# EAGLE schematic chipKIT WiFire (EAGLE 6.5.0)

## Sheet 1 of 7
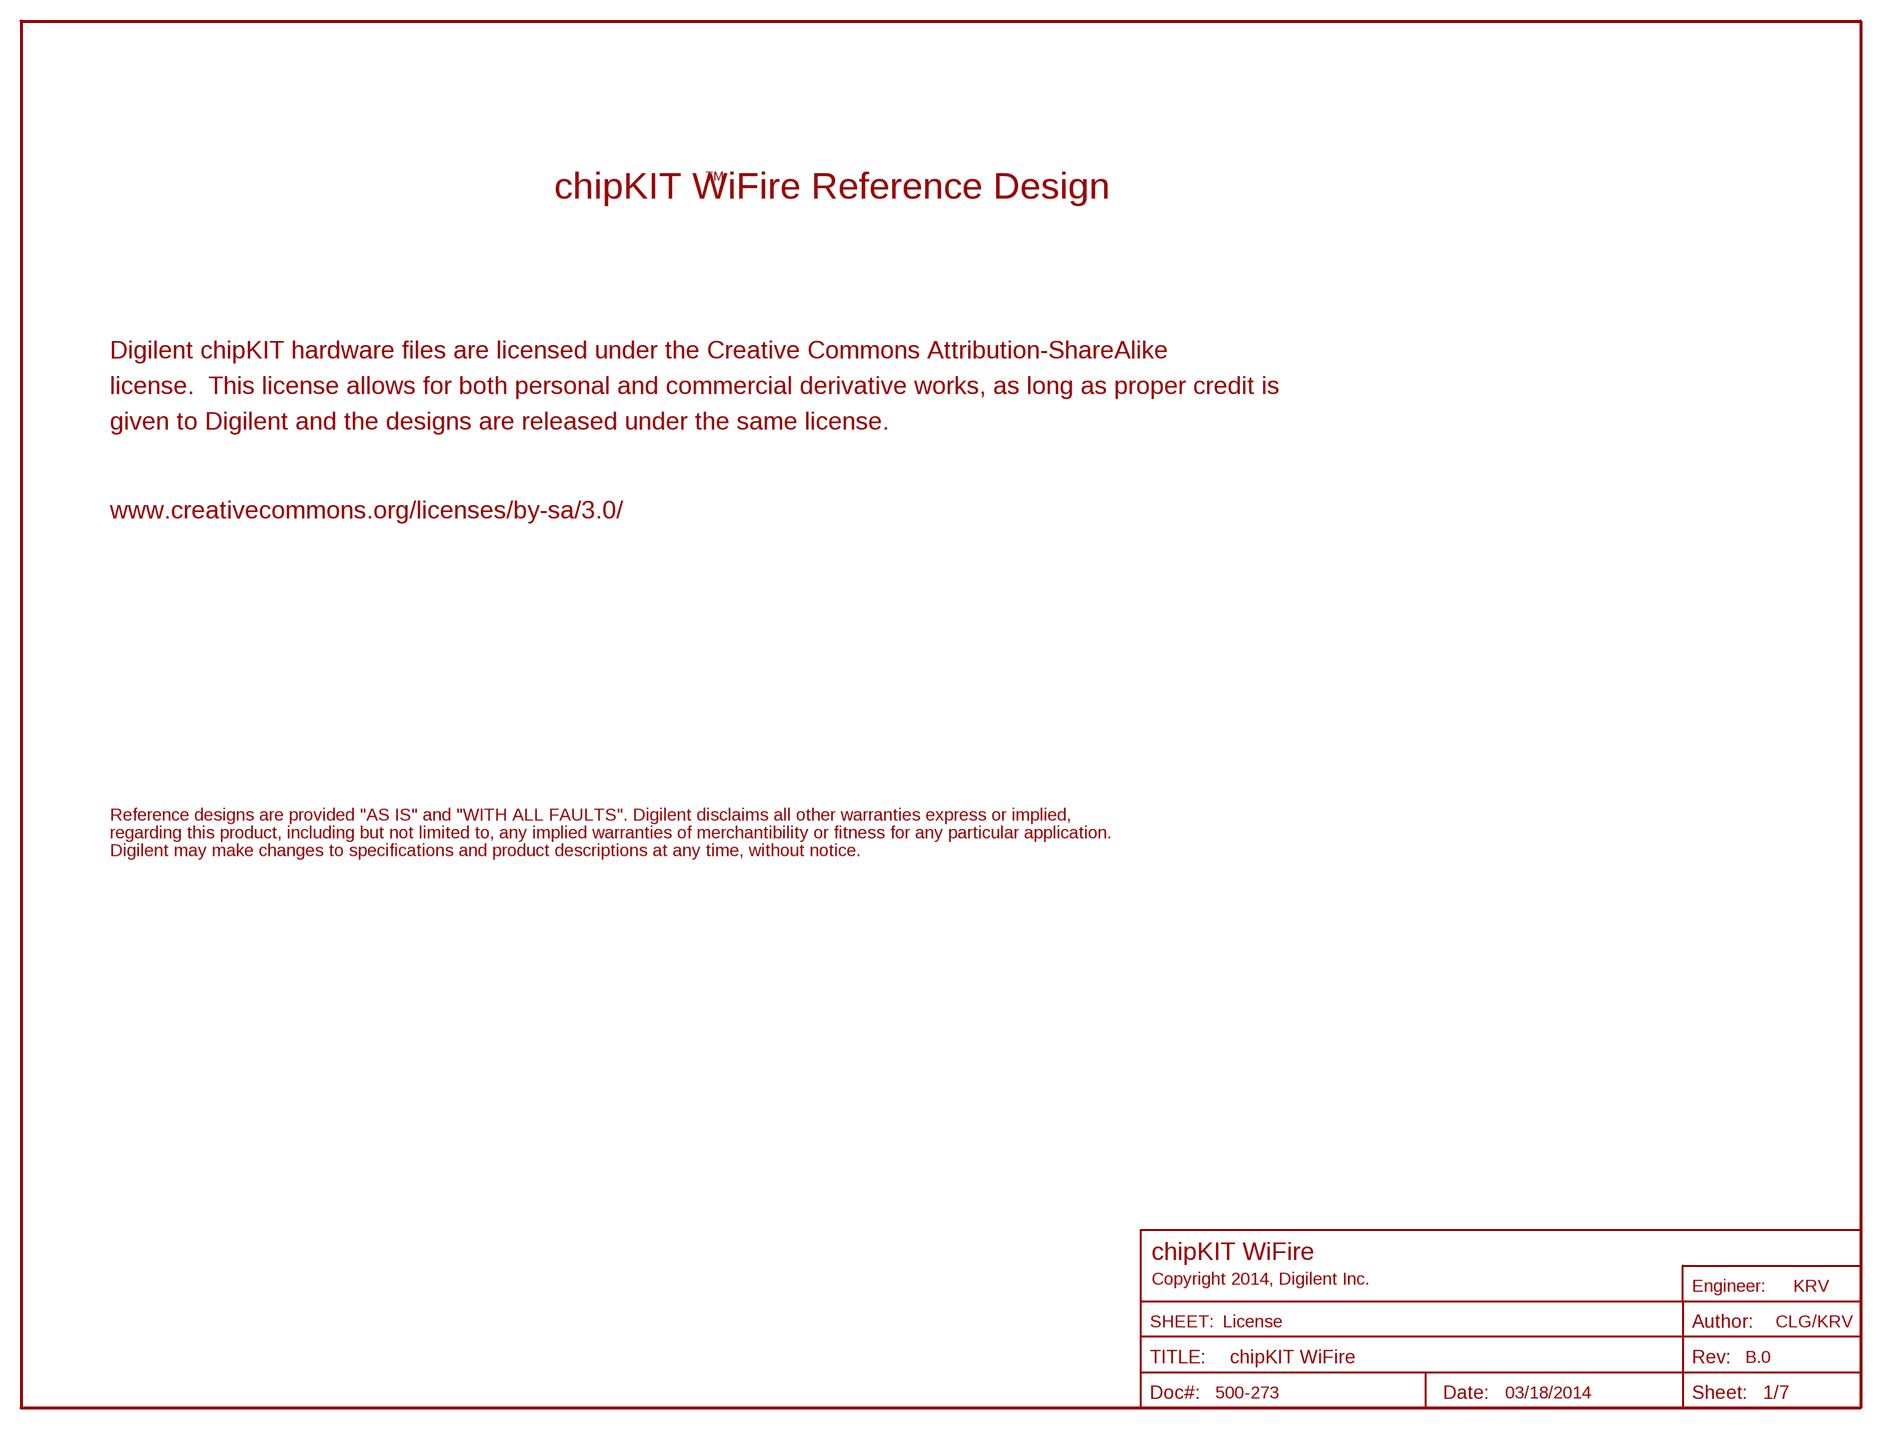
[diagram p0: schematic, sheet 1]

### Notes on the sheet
- TM
- chipKIT WiFire Reference Design
- Digilent chipKIT hardware files are licensed under the Creative Commons Attribution-ShareAlike
- license.  This license allows for both personal and commercial derivative works, as long as proper credit is
- given to Digilent and the designs are released under the same license.
- www.creativecommons.org/licenses/by-sa/3.0/
- Reference designs are provided "AS IS" and "WITH ALL FAULTS". Digilent disclaims all other warranties express or implied,
- regarding this product, including but not limited to, any implied warranties of merchantibility or fitness for any particular application.
- Digilent may make changes to specifications and product descriptions at any time, without notice.
- chipKIT WiFire
- Copyright 2014, Digilent Inc.
- KRV
- License | CLG/KRV
- B.0
- 500-273 | 03/18/2014

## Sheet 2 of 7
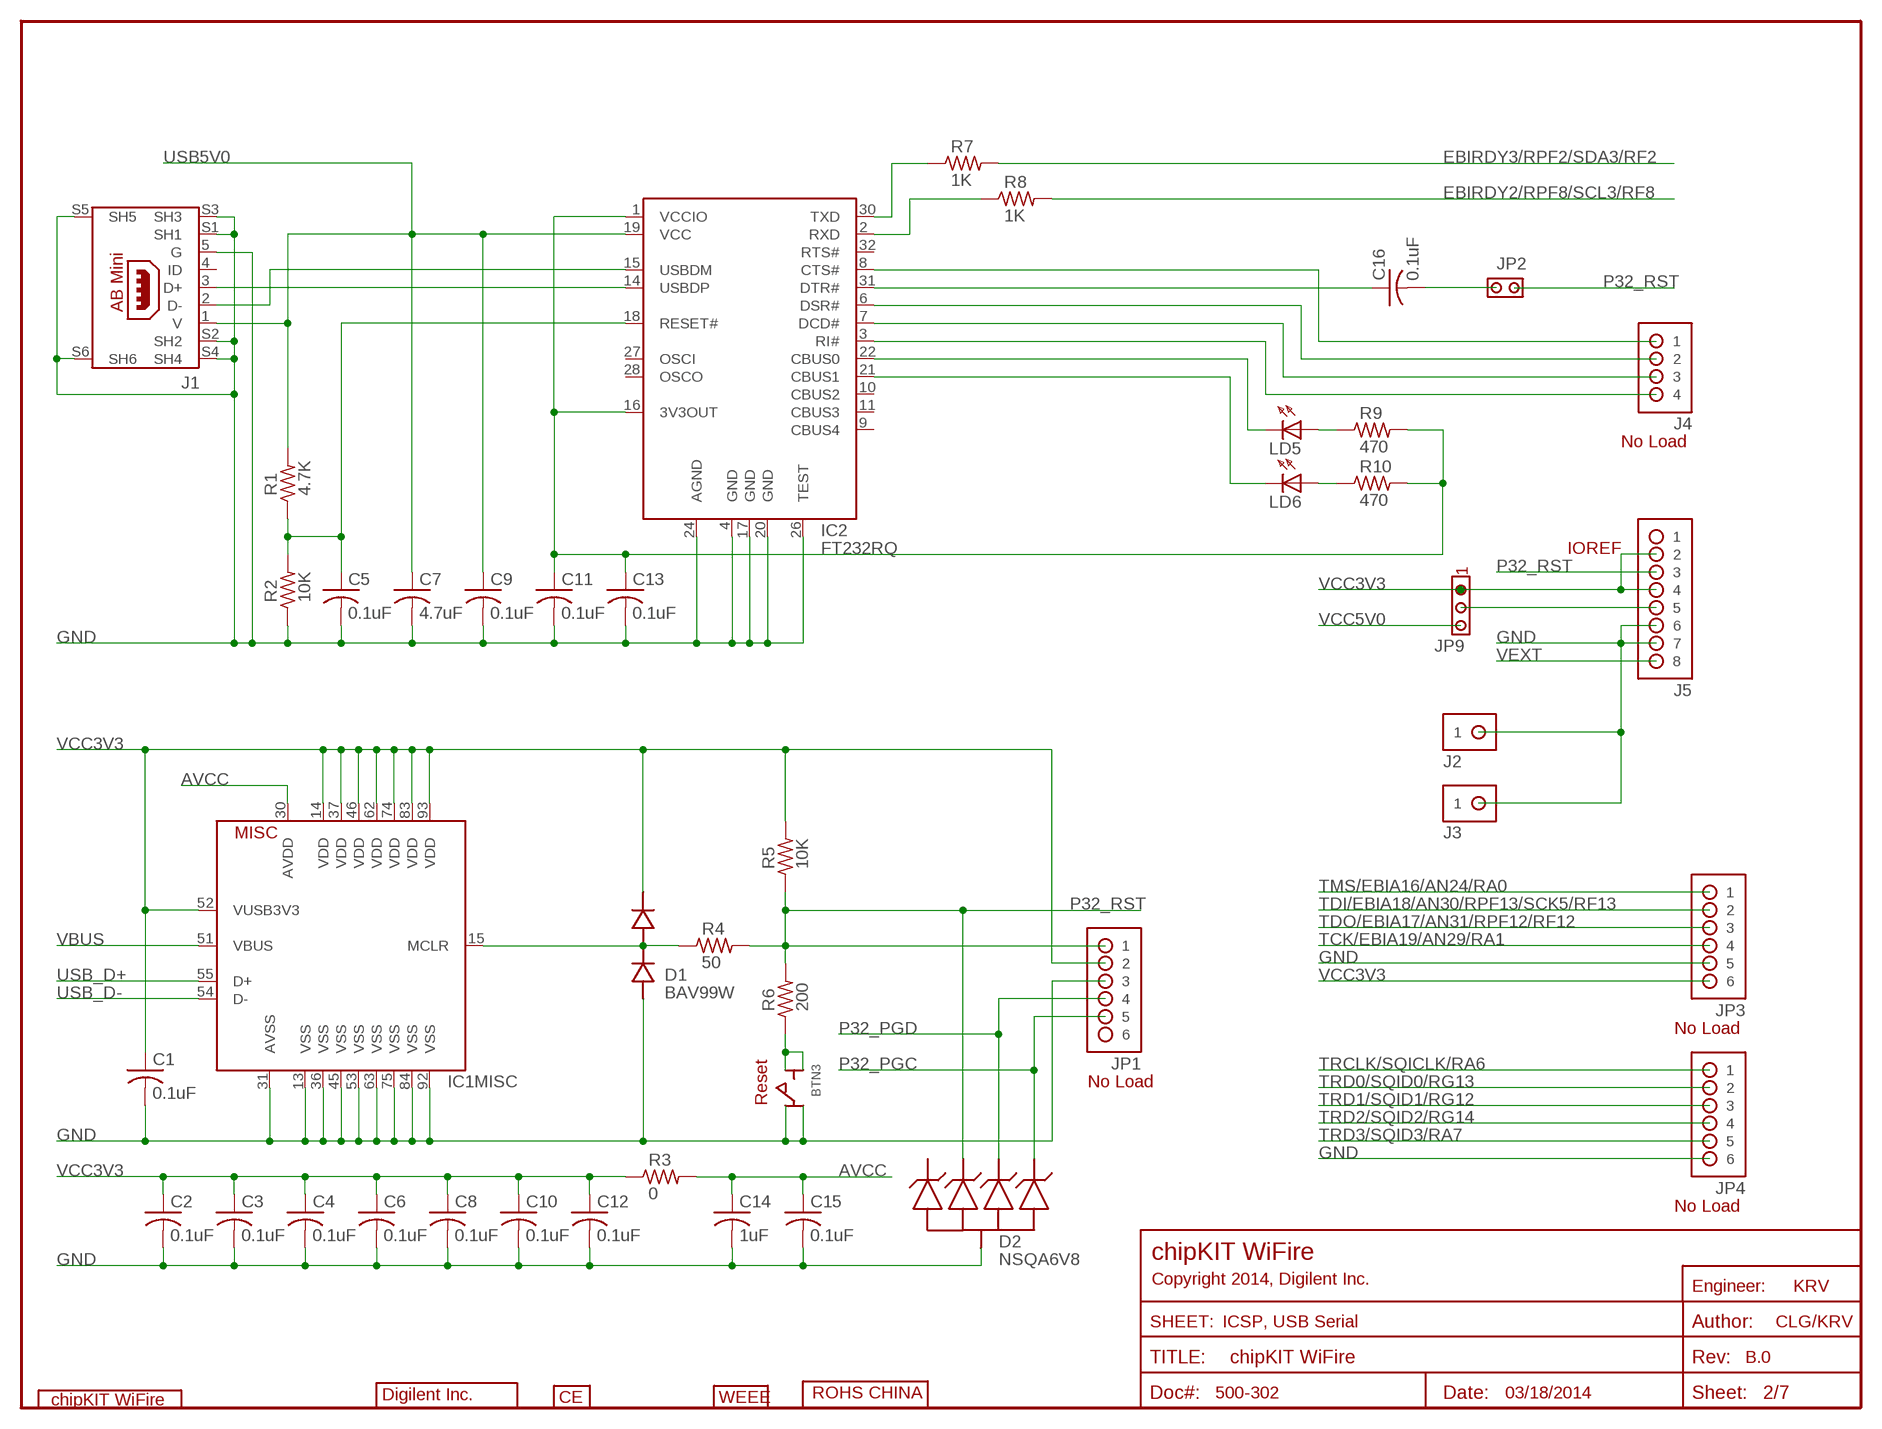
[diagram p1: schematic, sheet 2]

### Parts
BTN3  SW-P8008  [SW-P8008]
C1  0.1uF  CAP-S0402S  [C0402S]
C2  0.1uF  CAP-S0402S  [C0402S]
C3  0.1uF  CAP-S0402S  [C0402S]
C4  0.1uF  CAP-S0402S  [C0402S]
C5  0.1uF  CAP-S0402S  [C0402S]
C6  0.1uF  CAP-S0402S  [C0402S]
C7  4.7uF  CAP-S0603S  [C0603S]
C8  0.1uF  CAP-S0402S  [C0402S]
C9  0.1uF  CAP-S0402S  [C0402S]
C10  0.1uF  CAP-S0402S  [C0402S]
C11  0.1uF  CAP-S0402S  [C0402S]
C12  0.1uF  CAP-S0402S  [C0402S]
C13  0.1uF  CAP-S0402S  [C0402S]
C14  1uF  CAP-S0402S  [C0402S]
C15  0.1uF  CAP-S0402S  [C0402S]
C16  0.1uF  CAP-S0402S  [C0402S]
D1  BAV99W  [SOT-323]
D2  NSQA6V8  [SOT-323-5]
IC1  PIC32MZ2048ECG100-PT  PIC32MZECX100-PT  [TQ100-PT]
IC2  FT232RQ  [QFN32]
J1  KMAB-SMT-5S  USB-AB-MINI  [USB-AB-MINI]
J2  ST. Male  HDR-1X1  [HDR-1X1]
J3  ST. Male  HDR-1X1  [HDR-1X1]
J4  No Load  HDR-1X4  [HDR-1X4]
J5  ST. Female  HDR-1X8  [HDR-1X8]
JP1  No Load  HDR-1X6-OFFSET  [HDR-1X6_OFFSET]
JP2  ST. Male  JPR-1X2  [JPR-1X2]
JP3  No Load  HDR-1X6-OFFSET  [HDR-1X6_OFFSET]
JP4  No Load  HDR-1X6-OFFSET  [HDR-1X6_OFFSET]
JP9  JPR-1X3  [JPR-1X3]
LD5  Red  LED-S0603S  [D0603S]
LD6  Red  LED-S0603S  [D0603S]
LOGO1  DIGILENT_INC-BT-1000  [DIGILENT_BEYOND_1000_LOGO]
LOGO2  CE  [CE_LOGO]
LOGO3  WEEE-S  [WEEE_LOGO]
LOGO4  ROHS-CHINA  [ROHS_CHINA_LOGO]
R1  4.7K  RES-S0402S  [R0402S]
R2  10K  RES-S0402S  [R0402S]
R3  0  RES-S0603S  [R0603S]
R4  50  RES-S0402S  [R0402S]
R5  10K  RES-S0402S  [R0402S]
R6  200  RES-S0402S  [R0402S]
R7  1K  RES-S0402S  [R0402S]
R8  1K  RES-S0402S  [R0402S]
R9  470  RES-S0402S  [R0402S]
R10  470  RES-S0402S  [R0402S]
U$1  CHIPKIT_WIFIRE_LOGO  [CHIPKIT_WIFIRE_LOGO]

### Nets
AVCC: C14.1 C15.1 IC1.30(MISC:AVDD) R3.2
EBIRDY2/RPF8/SCL3/RF8: R8.2 ; also sheet 3,5
EBIRDY3/RPF2/SDA3/RF2: R7.2 ; also sheet 3,5
FT3V3: C11.1 C13.1 IC2.1(VCCIO) IC2.16(3V3OUT) R9.2 R10.2
GND: BTN3.1A BTN3.2A C1.2 C2.2 C3.2 C4.2 C5.2 C6.2 C7.2 C8.2 C9.2 C10.2 C11.2 C12.2 C13.2 C14.2 C15.2 D1.1(CAT) D2.2(COM) IC1.13(MISC:VSS) IC1.31(MISC:AVSS) IC1.36(MISC:VSS) IC1.45(MISC:VSS) IC1.53(MISC:VSS) IC1.63(MISC:VSS) IC1.75(MISC:VSS) IC1.84(MISC:VSS) IC1.92(MISC:VSS) IC2.4(GND) IC2.17(GND) IC2.20(GND) IC2.24(AGND) IC2.26(TEST) J1.5(G) J1.S1(SH1) J1.S2(SH2) J1.S3(SH3) J1.S4(SH4) J1.S5(SH5) J1.S6(SH6) J2.1 J3.1 J5.6 J5.7 JP1.3 JP3.5 JP4.6 R2.1 ; also sheet 3,4,5,6,7
N$14: C16.2 JP2.2
N$21: D1.3(COM) IC1.15(MISC:MCLR) R4.1
N$27: BTN3.1B BTN3.2B R6.1
N$33: IC2.15(USBDM) J1.2(D-)
N$37: IC2.14(USBDP) J1.3(D+)
N$41: IC2.30(TXD) R7.1
N$43: IC2.2(RXD) R8.1
N$47: C5.1 IC2.18(RESET#) R1.1 R2.2
N$52: IC2.8(CTS#) J4.1
N$53: C16.1 IC2.31(DTR#)
N$54: IC2.6(DSR#) J4.2
N$55: IC2.7(DCD#) J4.3
N$56: IC2.3(RI#) J4.4
N$57: IC2.22(CBUS0) LD5.C
N$58: IC2.21(CBUS1) LD6.C
N$59: LD5.A R9.1
N$60: LD6.A R10.1
P32_PGC: D2.5(D4) JP1.5 ; also sheet 4
P32_PGD: D2.4(D3) JP1.4 ; also sheet 4
P32_RST: D2.3(D2) J5.3 JP1.1 JP2.1 R4.2 R5.1 R6.2
TCK/EBIA19/AN29/RA1: JP3.4 ; also sheet 4
TDI/EBIA18/AN30/RPF13/SCK5/RF13: JP3.2 ; also sheet 5
TDO/EBIA17/AN31/RPF12/RF12: JP3.3 ; also sheet 5
TMS/EBIA16/AN24/RA0: JP3.1 ; also sheet 4
TRCLK/SQICLK/RA6: JP4.1 ; also sheet 4
TRD0/SQID0/RG13: JP4.2 ; also sheet 5
TRD1/SQID1/RG12: JP4.3 ; also sheet 5
TRD2/SQID2/RG14: JP4.4 ; also sheet 5
TRD3/SQID3/RA7: JP4.5 ; also sheet 4
USB5V0: C7.1 C9.1 IC2.19(VCC) J1.1(V) R1.2 ; also sheet 7
USB_D+: IC1.55(MISC:D+) ; also sheet 6
USB_D-: IC1.54(MISC:D-) ; also sheet 6
VBUS: IC1.51(MISC:VBUS) ; also sheet 6,7
VCC3V3: C1.1 C2.1 C3.1 C4.1 C6.1 C8.1 C10.1 C12.1 D1.2(AN) IC1.14(MISC:VDD) IC1.37(MISC:VDD) IC1.46(MISC:VDD) IC1.52(MISC:VUSB3V3) IC1.62(MISC:VDD) IC1.74(MISC:VDD) IC1.83(MISC:VDD) IC1.93(MISC:VDD) J5.2 J5.4 JP1.2 JP3.6 JP9.1 R3.1 R5.2 ; also sheet 4,5,6,7
VCC5V0: JP9.3 ; also sheet 6,7
VCCSHIELD: J5.5 JP9.2
VEXT: J5.8 ; also sheet 7
Unconnected: D2.1(D1) IC2.9(CBUS4) IC2.10(CBUS2) IC2.11(CBUS3) IC2.27(OSCI) IC2.28(OSCO) IC2.32(RTS#) J1.4(ID) J5.1 JP1.6

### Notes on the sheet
- No Load
- IOREF
- No Load
- No Load
- Reset
- No Load
- chipKIT WiFire
- Copyright 2014, Digilent Inc.
- KRV
- ICSP, USB Serial | CLG/KRV
- B.0
- 500-302 | 03/18/2014

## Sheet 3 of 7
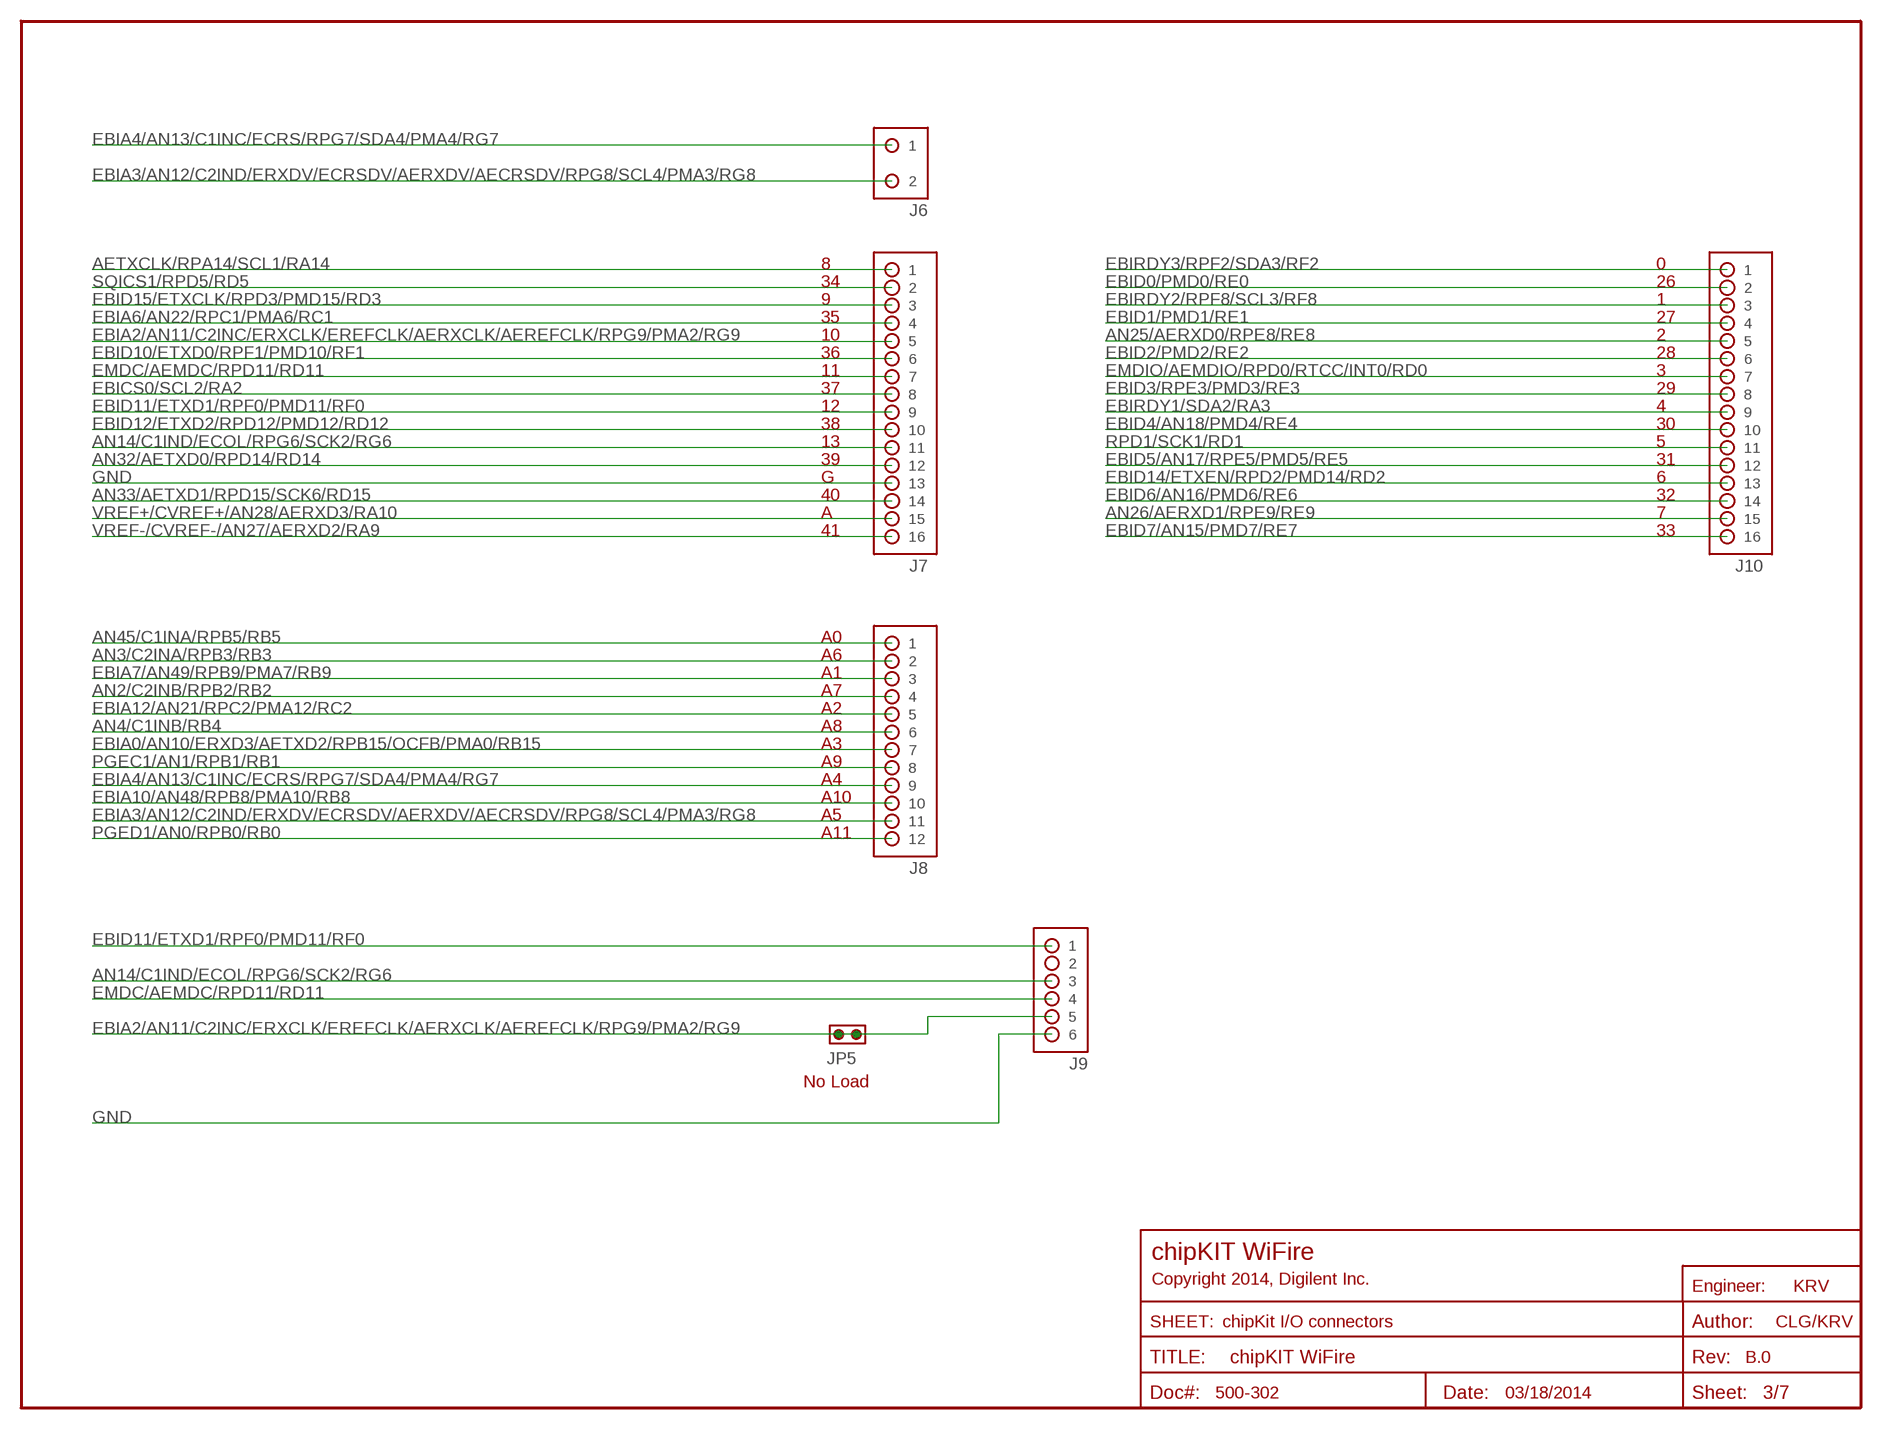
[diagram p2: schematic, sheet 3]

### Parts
J6  ST. Female  HDR-1X2  [HDR-1X2]
J7  ST. Female  HDR-2X8  [HDR-2X8]
J8  ST. Female  HDR-2X6  [HDR-2X6]
J9  ST. Male  HDR-2X3  [HDR-2X3]
J10  ST. Female  HDR-2X8  [HDR-2X8]
JP5  No Load  JPR-1X2  [JPR-1X2]

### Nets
AETXCLK/RPA14/SCL1/RA14: J7.1 ; also sheet 4,6
AN2/C2INB/RPB2/RB2: J8.4 ; also sheet 4
AN3/C2INA/RPB3/RB3: J8.2 ; also sheet 4
AN4/C1INB/RB4: J8.6 ; also sheet 4
AN14/C1IND/ECOL/RPG6/SCK2/RG6: J7.11 J9.3 ; also sheet 5,6
AN25/AERXD0/RPE8/RE8: J10.5 ; also sheet 5
AN26/AERXD1/RPE9/RE9: J10.15 ; also sheet 5
AN32/AETXD0/RPD14/RD14: J7.12 ; also sheet 5
AN33/AETXD1/RPD15/SCK6/RD15: J7.14 ; also sheet 5
AN45/C1INA/RPB5/RB5: J8.1 ; also sheet 4
EBIA0/AN10/ERXD3/AETXD2/RPB15/OCFB/PMA0/RB15: J8.7 ; also sheet 4
EBIA2/AN11/C2INC/ERXCLK/EREFCLK/AERXCLK/AEREFCLK/RPG9/PMA2/RG9: J7.5 J9.5 JP5.1 JP5.2 ; also sheet 5
EBIA3/AN12/C2IND/ERXDV/ECRSDV/AERXDV/AECRSDV/RPG8/SCL4/PMA3/RG8: J6.2 J8.11 ; also sheet 5
EBIA4/AN13/C1INC/ECRS/RPG7/SDA4/PMA4/RG7: J6.1 J8.9 ; also sheet 5
EBIA6/AN22/RPC1/PMA6/RC1: J7.4 ; also sheet 5
EBIA7/AN49/RPB9/PMA7/RB9: J8.3 ; also sheet 4
EBIA10/AN48/RPB8/PMA10/RB8: J8.10 ; also sheet 4
EBIA12/AN21/RPC2/PMA12/RC2: J8.5 ; also sheet 5
EBICS0/SCL2/RA2: J7.8 ; also sheet 4
EBID0/PMD0/RE0: J10.2 ; also sheet 5
EBID1/PMD1/RE1: J10.4 ; also sheet 5
EBID2/PMD2/RE2: J10.6 ; also sheet 5
EBID3/RPE3/PMD3/RE3: J10.8 ; also sheet 5
EBID4/AN18/PMD4/RE4: J10.10 ; also sheet 5
EBID5/AN17/RPE5/PMD5/RE5: J10.12 ; also sheet 5
EBID6/AN16/PMD6/RE6: J10.14 ; also sheet 5
EBID7/AN15/PMD7/RE7: J10.16 ; also sheet 5
EBID10/ETXD0/RPF1/PMD10/RF1: J7.6 ; also sheet 5
EBID11/ETXD1/RPF0/PMD11/RF0: J7.9 J9.1 ; also sheet 5
EBID12/ETXD2/RPD12/PMD12/RD12: J7.10 ; also sheet 5
EBID14/ETXEN/RPD2/PMD14/RD2: J10.13 ; also sheet 5
EBID15/ETXCLK/RPD3/PMD15/RD3: J7.3 ; also sheet 5
EBIRDY1/SDA2/RA3: J10.9 ; also sheet 4
EBIRDY2/RPF8/SCL3/RF8: J10.3 ; also sheet 2,5
EBIRDY3/RPF2/SDA3/RF2: J10.1 ; also sheet 2,5
EMDC/AEMDC/RPD11/RD11: J7.7 J9.4 ; also sheet 5
EMDIO/AEMDIO/RPD0/RTCC/INT0/RD0: J10.7 ; also sheet 5
GND: J7.13 J9.6 ; also sheet 2,4,5,6,7
PGEC1/AN1/RPB1/RB1: J8.8 ; also sheet 4
PGED1/AN0/RPB0/RB0: J8.12 ; also sheet 4,6
RPD1/SCK1/RD1: J10.11 ; also sheet 5
SQICS1/RPD5/RD5: J7.2 ; also sheet 5
VREF+/CVREF+/AN28/AERXD3/RA10: J7.15 ; also sheet 4
VREF-/CVREF-/AN27/AERXD2/RA9: J7.16 ; also sheet 4
Unconnected: J9.2

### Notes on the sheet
- 8 | 0
- 34 | 26
- 9 | 1
- 35 | 27
- 10 | 2
- 36 | 28
- 11 | 3
- 37 | 29
- 12 | 4
- 38 | 30
- 13 | 5
- 39 | 31
- G | 6
- 40 | 32
- A | 7
- 41 | 33
- A0
- A6
- A1
- A7
- A2
- A8
- A3
- A9
- A4
- A10
- A5
- A11
- No Load
- chipKIT WiFire
- Copyright 2014, Digilent Inc.
- KRV
- chipKit I/O connectors | CLG/KRV
- B.0
- 500-302 | 03/18/2014

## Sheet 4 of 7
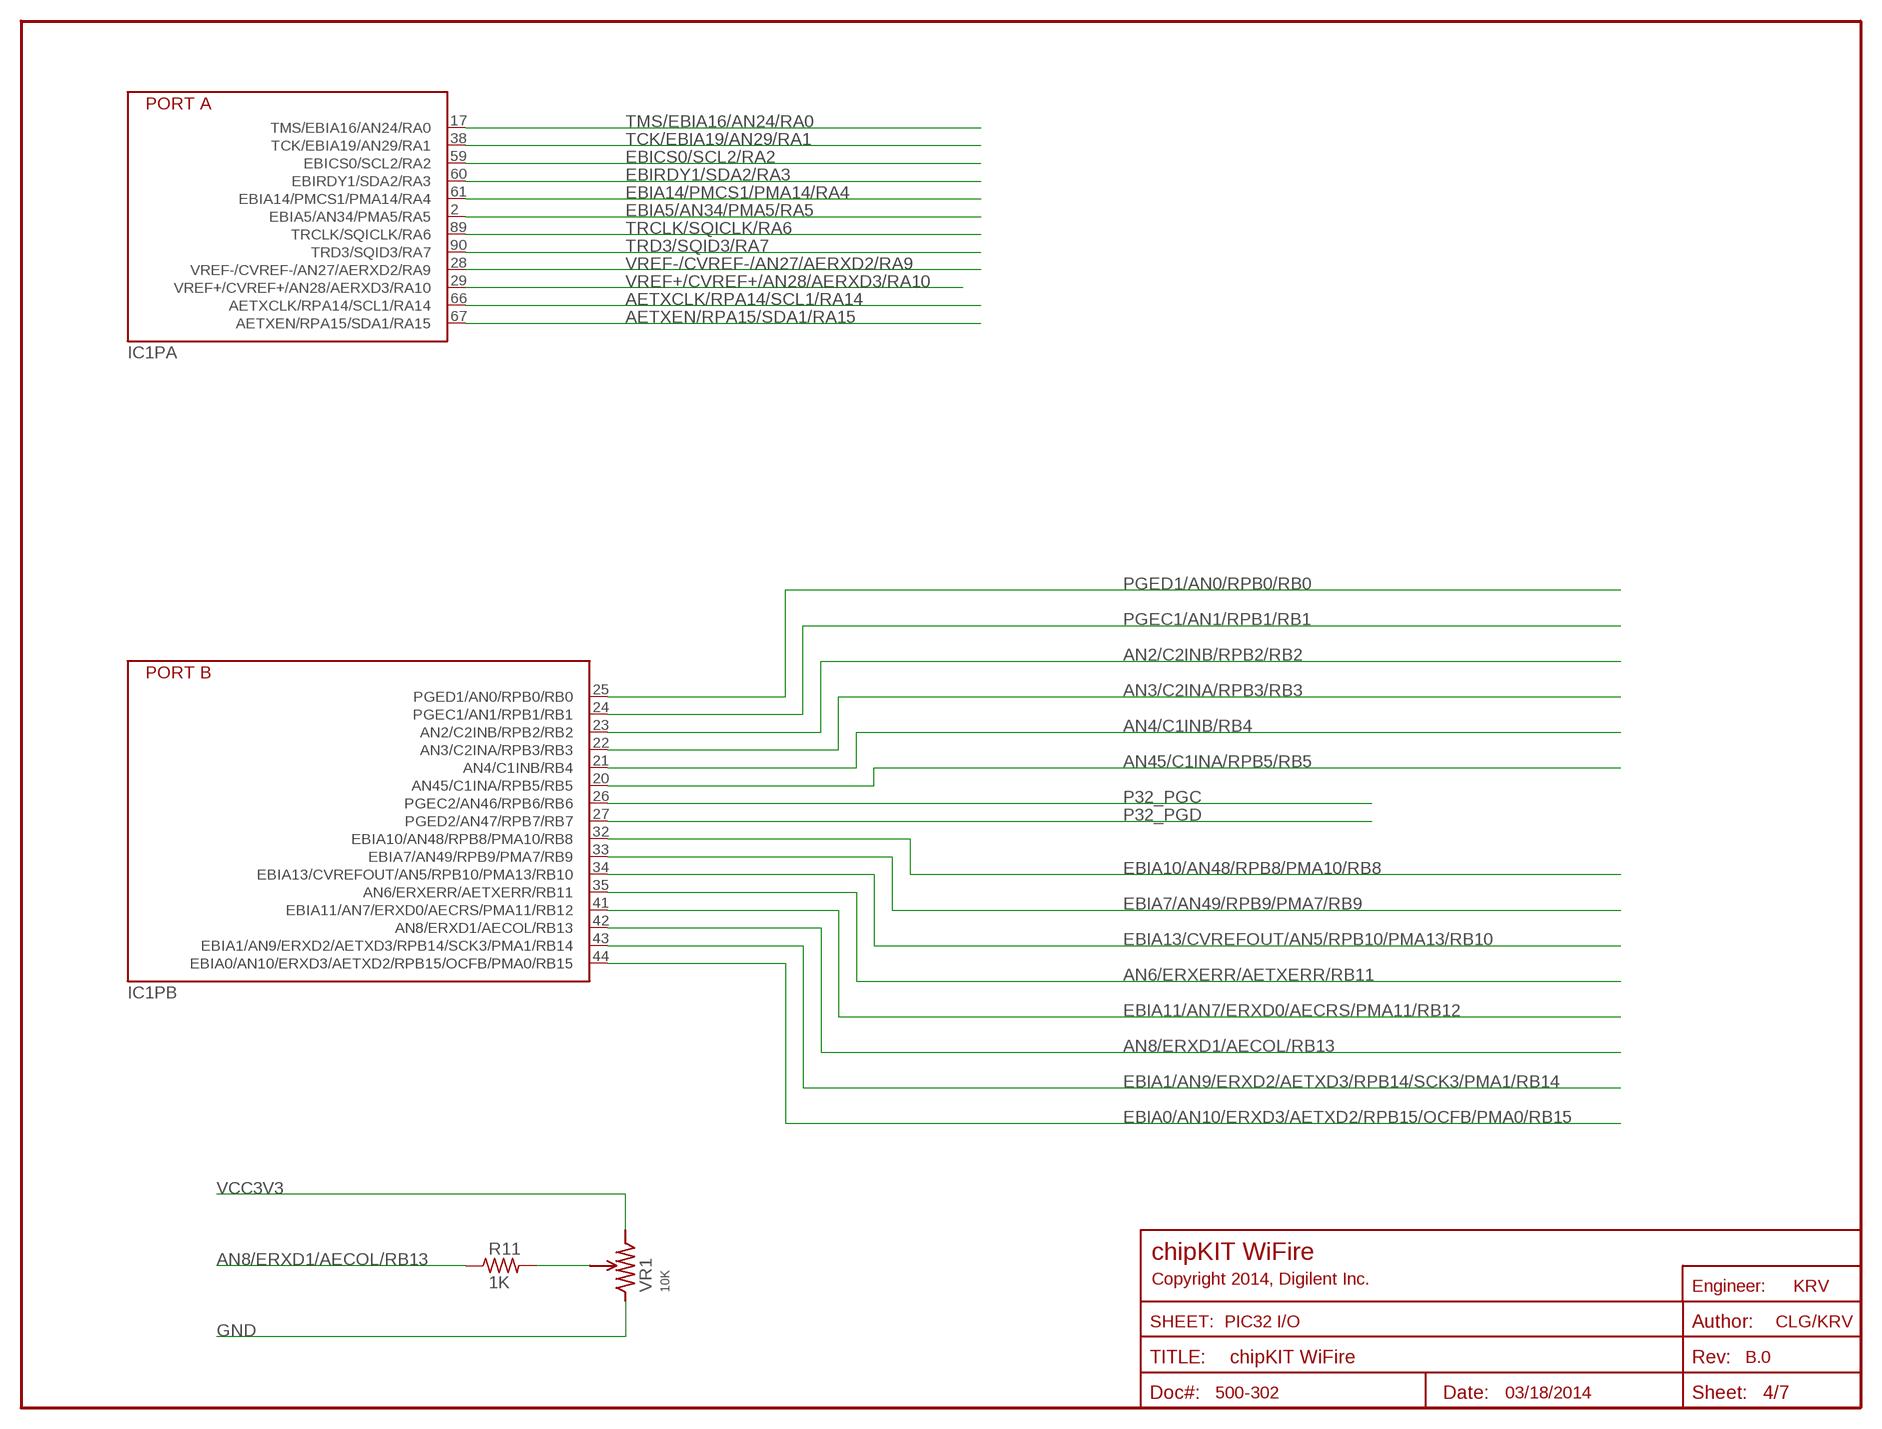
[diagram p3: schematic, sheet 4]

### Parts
R11  1K  RES-S0402S  [R0402S]
VR1  10K  POT-3352T  [BOURNS-3352T]

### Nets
AETXCLK/RPA14/SCL1/RA14: IC1.66(PA:AETXCLK/RPA14/SCL1/RA14) ; also sheet 3,6
AETXEN/RPA15/SDA1/RA15: IC1.67(PA:AETXEN/RPA15/SDA1/RA15) ; also sheet 6
AN2/C2INB/RPB2/RB2: IC1.23(PB:AN2/C2INB/RPB2/RB2) ; also sheet 3
AN3/C2INA/RPB3/RB3: IC1.22(PB:AN3/C2INA/RPB3/RB3) ; also sheet 3
AN4/C1INB/RB4: IC1.21(PB:AN4/C1INB/RB4) ; also sheet 3
AN6/ERXERR/AETXERR/RB11: IC1.35(PB:AN6/ERXERR/AETXERR/RB11) ; also sheet 6
AN8/ERXD1/AECOL/RB13: IC1.42(PB:AN8/ERXD1/AECOL/RB13) R11.1
AN45/C1INA/RPB5/RB5: IC1.20(PB:AN45/C1INA/RPB5/RB5) ; also sheet 3
EBIA0/AN10/ERXD3/AETXD2/RPB15/OCFB/PMA0/RB15: IC1.44(PB:EBIA0/AN10/ERXD3/AETXD2/RPB15/OCFB/PMA0/RB15) ; also sheet 3
EBIA1/AN9/ERXD2/AETXD3/RPB14/SCK3/PMA1/RB14: IC1.43(PB:EBIA1/AN9/ERXD2/AETXD3/RPB14/SCK3/PMA1/RB14) ; also sheet 6
EBIA5/AN34/PMA5/RA5: IC1.2(PA:EBIA5/AN34/PMA5/RA5) ; also sheet 6
EBIA7/AN49/RPB9/PMA7/RB9: IC1.33(PB:EBIA7/AN49/RPB9/PMA7/RB9) ; also sheet 3
EBIA10/AN48/RPB8/PMA10/RB8: IC1.32(PB:EBIA10/AN48/RPB8/PMA10/RB8) ; also sheet 3
EBIA11/AN7/ERXD0/AECRS/PMA11/RB12: IC1.41(PB:EBIA11/AN7/ERXD0/AECRS/PMA11/RB12) ; also sheet 7
EBIA13/CVREFOUT/AN5/RPB10/PMA13/RB10: IC1.34(PB:EBIA13/CVREFOUT/AN5/RPB10/PMA13/RB10) ; also sheet 6
EBIA14/PMCS1/PMA14/RA4: IC1.61(PA:EBIA14/PMCS1/PMA14/RA4) ; also sheet 6
EBICS0/SCL2/RA2: IC1.59(PA:EBICS0/SCL2/RA2) ; also sheet 3
EBIRDY1/SDA2/RA3: IC1.60(PA:EBIRDY1/SDA2/RA3) ; also sheet 3
GND: VR1.1 ; also sheet 2,3,5,6,7
N$40: R11.2 VR1.2
P32_PGC: IC1.26(PB:PGEC2/AN46/RPB6/RB6) ; also sheet 2
P32_PGD: IC1.27(PB:PGED2/AN47/RPB7/RB7) ; also sheet 2
PGEC1/AN1/RPB1/RB1: IC1.24(PB:PGEC1/AN1/RPB1/RB1) ; also sheet 3
PGED1/AN0/RPB0/RB0: IC1.25(PB:PGED1/AN0/RPB0/RB0) ; also sheet 3,6
TCK/EBIA19/AN29/RA1: IC1.38(PA:TCK/EBIA19/AN29/RA1) ; also sheet 2
TMS/EBIA16/AN24/RA0: IC1.17(PA:TMS/EBIA16/AN24/RA0) ; also sheet 2
TRCLK/SQICLK/RA6: IC1.89(PA:TRCLK/SQICLK/RA6) ; also sheet 2
TRD3/SQID3/RA7: IC1.90(PA:TRD3/SQID3/RA7) ; also sheet 2
VCC3V3: VR1.3 ; also sheet 2,5,6,7
VREF+/CVREF+/AN28/AERXD3/RA10: IC1.29(PA:VREF+/CVREF+/AN28/AERXD3/RA10) ; also sheet 3
VREF-/CVREF-/AN27/AERXD2/RA9: IC1.28(PA:VREF-/CVREF-/AN27/AERXD2/RA9) ; also sheet 3

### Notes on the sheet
- chipKIT WiFire
- Copyright 2014, Digilent Inc.
- KRV
- PIC32 I/O | CLG/KRV
- B.0
- 500-302 | 03/18/2014

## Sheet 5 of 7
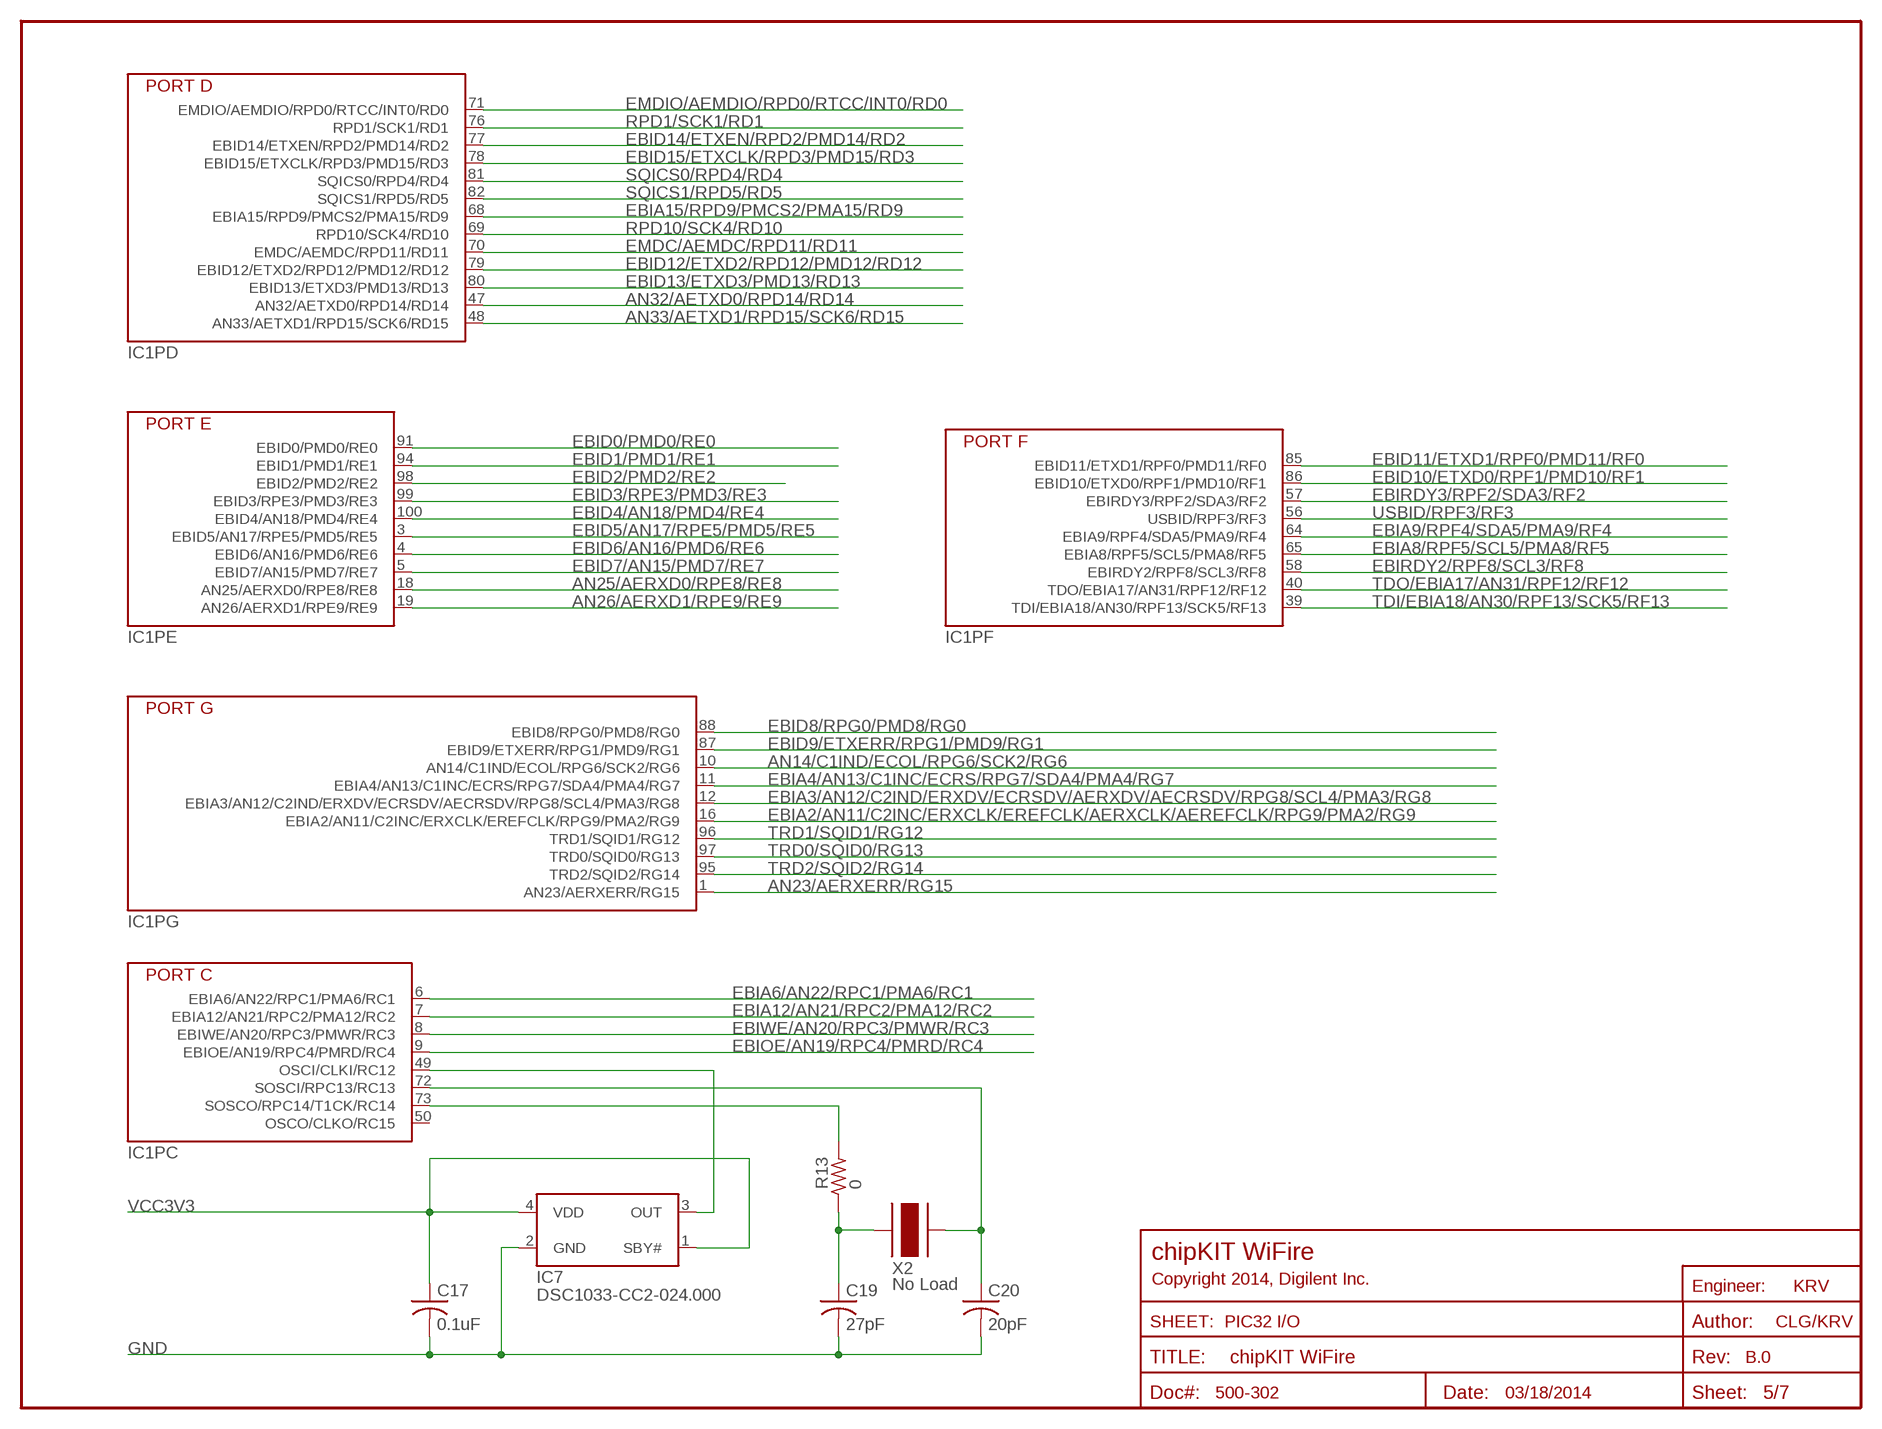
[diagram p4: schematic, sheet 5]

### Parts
C17  0.1uF  CAP-S0402S  [C0402S]
C19  27pF  CAP-S0402S  [C0402S]
C20  20pF  CAP-S0402S  [C0402S]
IC7  DSC1033-CC2-024.000  DSC1033-C  [DSC1033-C]
R13  0  RES-S0402S  [R0402S]
X2  No Load  XTAL-T38  [XT-T38]

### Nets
AN14/C1IND/ECOL/RPG6/SCK2/RG6: IC1.10(PG:AN14/C1IND/ECOL/RPG6/SCK2/RG6) ; also sheet 3,6
AN23/AERXERR/RG15: IC1.1(PG:AN23/AERXERR/RG15) ; also sheet 6
AN25/AERXD0/RPE8/RE8: IC1.18(PE:AN25/AERXD0/RPE8/RE8) ; also sheet 3
AN26/AERXD1/RPE9/RE9: IC1.19(PE:AN26/AERXD1/RPE9/RE9) ; also sheet 3
AN32/AETXD0/RPD14/RD14: IC1.47(PD:AN32/AETXD0/RPD14/RD14) ; also sheet 3
AN33/AETXD1/RPD15/SCK6/RD15: IC1.48(PD:AN33/AETXD1/RPD15/SCK6/RD15) ; also sheet 3
EBIA2/AN11/C2INC/ERXCLK/EREFCLK/AERXCLK/AEREFCLK/RPG9/PMA2/RG9: IC1.16(PG:EBIA2/AN11/C2INC/ERXCLK/EREFCLK/RPG9/PMA2/RG9) ; also sheet 3
EBIA3/AN12/C2IND/ERXDV/ECRSDV/AERXDV/AECRSDV/RPG8/SCL4/PMA3/RG8: IC1.12(PG:EBIA3/AN12/C2IND/ERXDV/ECRSDV/AECRSDV/RPG8/SCL4/PMA3/RG8) ; also sheet 3
EBIA4/AN13/C1INC/ECRS/RPG7/SDA4/PMA4/RG7: IC1.11(PG:EBIA4/AN13/C1INC/ECRS/RPG7/SDA4/PMA4/RG7) ; also sheet 3
EBIA6/AN22/RPC1/PMA6/RC1: IC1.6(PC:EBIA6/AN22/RPC1/PMA6/RC1) ; also sheet 3
EBIA8/RPF5/SCL5/PMA8/RF5: IC1.65(PF:EBIA8/RPF5/SCL5/PMA8/RF5) ; also sheet 6
EBIA9/RPF4/SDA5/PMA9/RF4: IC1.64(PF:EBIA9/RPF4/SDA5/PMA9/RF4) ; also sheet 6
EBIA12/AN21/RPC2/PMA12/RC2: IC1.7(PC:EBIA12/AN21/RPC2/PMA12/RC2) ; also sheet 3
EBIA15/RPD9/PMCS2/PMA15/RD9: IC1.68(PD:EBIA15/RPD9/PMCS2/PMA15/RD9) ; also sheet 6
EBID0/PMD0/RE0: IC1.91(PE:EBID0/PMD0/RE0) ; also sheet 3
EBID1/PMD1/RE1: IC1.94(PE:EBID1/PMD1/RE1) ; also sheet 3
EBID2/PMD2/RE2: IC1.98(PE:EBID2/PMD2/RE2) ; also sheet 3
EBID3/RPE3/PMD3/RE3: IC1.99(PE:EBID3/RPE3/PMD3/RE3) ; also sheet 3
EBID4/AN18/PMD4/RE4: IC1.100(PE:EBID4/AN18/PMD4/RE4) ; also sheet 3
EBID5/AN17/RPE5/PMD5/RE5: IC1.3(PE:EBID5/AN17/RPE5/PMD5/RE5) ; also sheet 3
EBID6/AN16/PMD6/RE6: IC1.4(PE:EBID6/AN16/PMD6/RE6) ; also sheet 3
EBID7/AN15/PMD7/RE7: IC1.5(PE:EBID7/AN15/PMD7/RE7) ; also sheet 3
EBID8/RPG0/PMD8/RG0: IC1.88(PG:EBID8/RPG0/PMD8/RG0) ; also sheet 6
EBID9/ETXERR/RPG1/PMD9/RG1: IC1.87(PG:EBID9/ETXERR/RPG1/PMD9/RG1) ; also sheet 6
EBID10/ETXD0/RPF1/PMD10/RF1: IC1.86(PF:EBID10/ETXD0/RPF1/PMD10/RF1) ; also sheet 3
EBID11/ETXD1/RPF0/PMD11/RF0: IC1.85(PF:EBID11/ETXD1/RPF0/PMD11/RF0) ; also sheet 3
EBID12/ETXD2/RPD12/PMD12/RD12: IC1.79(PD:EBID12/ETXD2/RPD12/PMD12/RD12) ; also sheet 3
EBID13/ETXD3/PMD13/RD13: IC1.80(PD:EBID13/ETXD3/PMD13/RD13) ; also sheet 7
EBID14/ETXEN/RPD2/PMD14/RD2: IC1.77(PD:EBID14/ETXEN/RPD2/PMD14/RD2) ; also sheet 3
EBID15/ETXCLK/RPD3/PMD15/RD3: IC1.78(PD:EBID15/ETXCLK/RPD3/PMD15/RD3) ; also sheet 3
EBIOE/AN19/RPC4/PMRD/RC4: IC1.9(PC:EBIOE/AN19/RPC4/PMRD/RC4) ; also sheet 6
EBIRDY2/RPF8/SCL3/RF8: IC1.58(PF:EBIRDY2/RPF8/SCL3/RF8) ; also sheet 2,3
EBIRDY3/RPF2/SDA3/RF2: IC1.57(PF:EBIRDY3/RPF2/SDA3/RF2) ; also sheet 2,3
EBIWE/AN20/RPC3/PMWR/RC3: IC1.8(PC:EBIWE/AN20/RPC3/PMWR/RC3) ; also sheet 6
EMDC/AEMDC/RPD11/RD11: IC1.70(PD:EMDC/AEMDC/RPD11/RD11) ; also sheet 3
EMDIO/AEMDIO/RPD0/RTCC/INT0/RD0: IC1.71(PD:EMDIO/AEMDIO/RPD0/RTCC/INT0/RD0) ; also sheet 3
GND: C17.2 C19.2 C20.2 IC7.2(GND) ; also sheet 2,3,4,6,7
N$17: IC1.49(PC:OSCI/CLKI/RC12) IC7.3(OUT)
N$18: C20.1 IC1.72(PC:SOSCI/RPC13/RC13) X2.2
N$19: IC1.73(PC:SOSCO/RPC14/T1CK/RC14) R13.2
N$20: C19.1 R13.1 X2.1
RPD1/SCK1/RD1: IC1.76(PD:RPD1/SCK1/RD1) ; also sheet 3
RPD10/SCK4/RD10: IC1.69(PD:RPD10/SCK4/RD10) ; also sheet 6
SQICS0/RPD4/RD4: IC1.81(PD:SQICS0/RPD4/RD4) ; also sheet 6
SQICS1/RPD5/RD5: IC1.82(PD:SQICS1/RPD5/RD5) ; also sheet 3
TDI/EBIA18/AN30/RPF13/SCK5/RF13: IC1.39(PF:TDI/EBIA18/AN30/RPF13/SCK5/RF13) ; also sheet 2
TDO/EBIA17/AN31/RPF12/RF12: IC1.40(PF:TDO/EBIA17/AN31/RPF12/RF12) ; also sheet 2
TRD0/SQID0/RG13: IC1.97(PG:TRD0/SQID0/RG13) ; also sheet 2
TRD1/SQID1/RG12: IC1.96(PG:TRD1/SQID1/RG12) ; also sheet 2
TRD2/SQID2/RG14: IC1.95(PG:TRD2/SQID2/RG14) ; also sheet 2
USBID/RPF3/RF3: IC1.56(PF:USBID/RPF3/RF3) ; also sheet 6
VCC3V3: C17.1 IC7.1(SBY#) IC7.4(VDD) ; also sheet 2,4,6,7
Unconnected: IC1.50(PC:OSCO/CLKO/RC15)

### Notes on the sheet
- chipKIT WiFire
- Copyright 2014, Digilent Inc.
- KRV
- PIC32 I/O | CLG/KRV
- B.0
- 500-302 | 03/18/2014

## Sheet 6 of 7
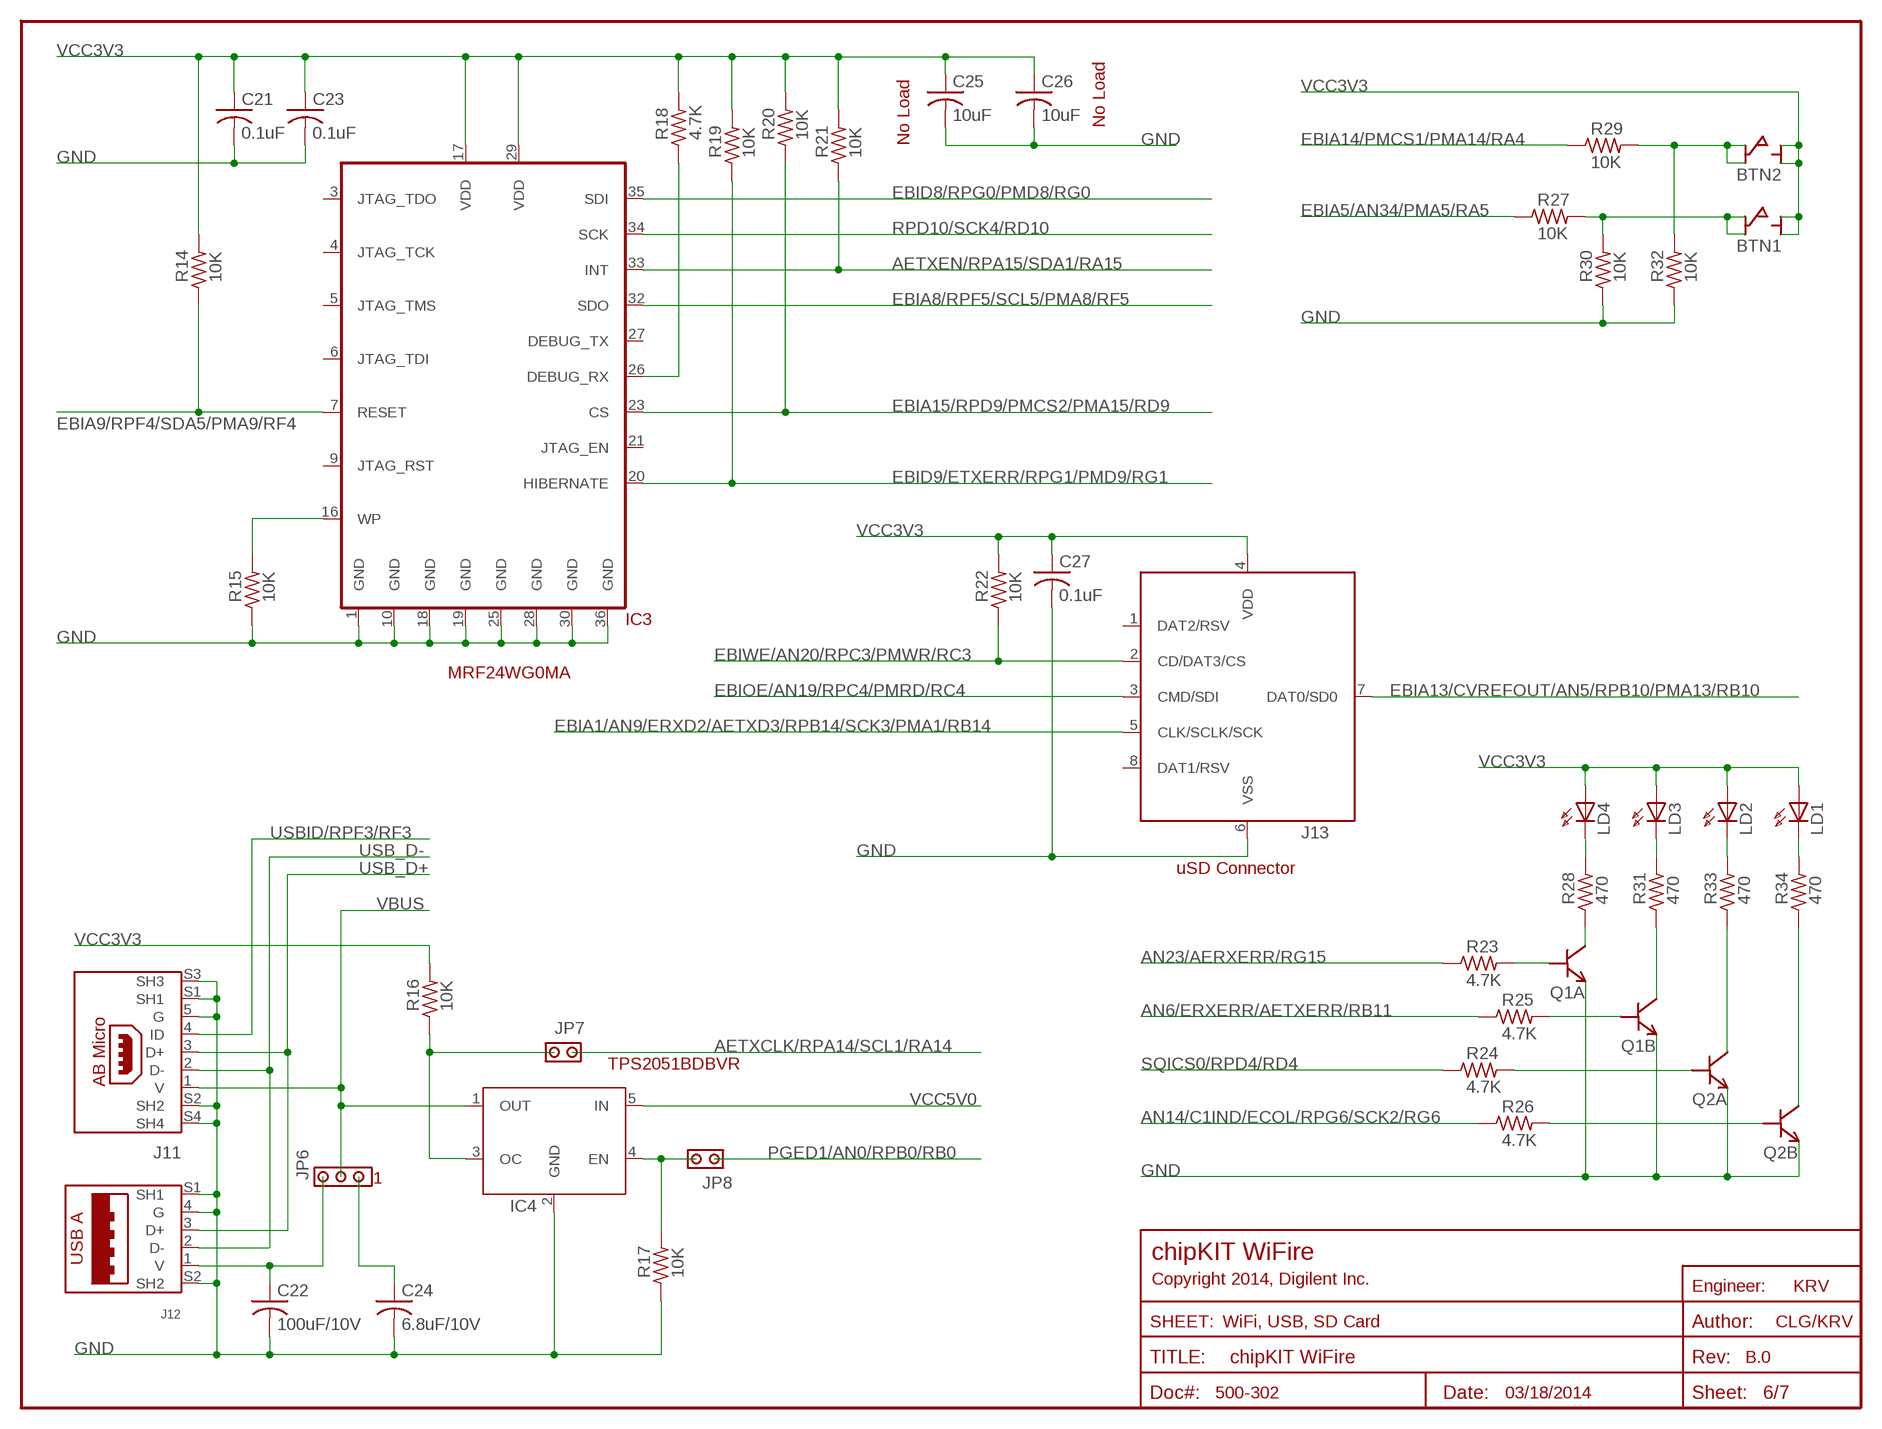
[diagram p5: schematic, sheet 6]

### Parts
BTN1  SW-P8008  [SW-P8008]
BTN2  SW-P8008  [SW-P8008]
C21  0.1uF  CAP-S0402S  [C0402S]
C22  100uF/10V  CAP-S1206S  [C1206S]
C23  0.1uF  CAP-S0402S  [C0402S]
C24  6.8uF/10V  CAP-S0603S  [C0603S]
C25  10uF  CAP-S0805S  [C0805S]
C26  10uF  CAP-S0805S  [C0805S]
C27  0.1uF  CAP-S0402S  [C0402S]
IC3  MRF24WG0MA  MRF24WB0MA  [MRF24WB0MA]
IC4  TPS2051BDBVR  TPS2041B-DBV  [SOT23-5]
J11  UMMCF-051MBCB-CF535  USB-AB-MICRO  [USB-AB-MICRO]
J12  KUSB-AS-1  USB-A  [USB-A]
J13  2908-05WB-MG  [2908-05WB-MG]
JP6  ST. Male  JPR-1X3  [JPR-1X3]
JP7  ST. Male  JPR-1X2  [JPR-1X2]
JP8  ST. Male  JPR-1X2  [JPR-1X2]
LD1  Green  LED-S0603S  [D0603S]
LD2  Green  LED-S0603S  [D0603S]
LD3  Green  LED-S0603S  [D0603S]
LD4  Green  LED-S0603S  [D0603S]
Q1  MBT3904DW1T1  [SOT-363]
Q2  MBT3904DW1T1  [SOT-363]
R14  10K  RES-S0402S  [R0402S]
R15  10K  RES-S0402S  [R0402S]
R16  10K  RES-S0402S  [R0402S]
R17  10K  RES-S0402S  [R0402S]
R18  4.7K  RES-S0402S  [R0402S]
R19  10K  RES-S0402S  [R0402S]
R20  10K  RES-S0402S  [R0402S]
R21  10K  RES-S0402S  [R0402S]
R22  10K  RES-S0402S  [R0402S]
R23  4.7K  RES-S0402S  [R0402S]
R24  4.7K  RES-S0402S  [R0402S]
R25  4.7K  RES-S0402S  [R0402S]
R26  4.7K  RES-S0402S  [R0402S]
R27  10K  RES-S0402S  [R0402S]
R28  470  RES-S0402S  [R0402S]
R29  10K  RES-S0402S  [R0402S]
R30  10K  RES-S0402S  [R0402S]
R31  470  RES-S0402S  [R0402S]
R32  10K  RES-S0402S  [R0402S]
R33  470  RES-S0402S  [R0402S]
R34  470  RES-S0402S  [R0402S]

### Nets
AETXCLK/RPA14/SCL1/RA14: JP7.2 ; also sheet 3,4
AETXEN/RPA15/SDA1/RA15: IC3.33(INT) R21.1 ; also sheet 4
AN6/ERXERR/AETXERR/RB11: R25.1 ; also sheet 4
AN14/C1IND/ECOL/RPG6/SCK2/RG6: R26.1 ; also sheet 3,5
AN23/AERXERR/RG15: R23.1 ; also sheet 5
EBIA1/AN9/ERXD2/AETXD3/RPB14/SCK3/PMA1/RB14: J13.5(CLK/SCLK/SCK) ; also sheet 4
EBIA5/AN34/PMA5/RA5: R27.1 ; also sheet 4
EBIA8/RPF5/SCL5/PMA8/RF5: IC3.32(SDO) ; also sheet 5
EBIA9/RPF4/SDA5/PMA9/RF4: IC3.7(RESET) R14.1 ; also sheet 5
EBIA13/CVREFOUT/AN5/RPB10/PMA13/RB10: J13.7(DAT0/SD0) ; also sheet 4
EBIA14/PMCS1/PMA14/RA4: R29.1 ; also sheet 4
EBIA15/RPD9/PMCS2/PMA15/RD9: IC3.23(CS) R20.1 ; also sheet 5
EBID8/RPG0/PMD8/RG0: IC3.35(SDI) ; also sheet 5
EBID9/ETXERR/RPG1/PMD9/RG1: IC3.20(HIBERNATE) R19.1 ; also sheet 5
EBIOE/AN19/RPC4/PMRD/RC4: J13.3(CMD/SDI) ; also sheet 5
EBIWE/AN20/RPC3/PMWR/RC3: J13.2(CD/DAT3/CS) R22.1 ; also sheet 5
GND: C21.2 C22.2 C23.2 C24.2 C25.2 C26.2 C27.2 IC3.1(GND) IC3.10(GND) IC3.18(GND) IC3.19(GND) IC3.25(GND) IC3.28(GND) IC3.30(GND) IC3.36(GND) IC4.2(GND) J11.5(G) J11.S1(SH1) J11.S2(SH2) J11.S3(SH3) J11.S4(SH4) J12.4(G) J12.S1(SH1) J12.S2(SH2) J13.6(VSS) Q1.1(B:E) Q1.4(A:E) Q2.1(B:E) Q2.4(A:E) R15.1 R17.1 R30.1 R32.1 ; also sheet 2,3,4,5,7
N$1: C24.1 JP6.1
N$22: Q2.5(A:B) R24.2
N$23: Q2.3(A:C) R33.1
N$25: IC4.3(OC) JP7.1 R16.1
N$26: LD2.C R33.2
N$28: LD1.C R34.2
N$29: IC3.26(DEBUG_RX) R18.1
N$31: Q2.2(B:B) R26.2
N$32: Q2.6(B:C) R34.1
N$45: IC3.16(WP) R15.2
N$51: LD3.C R31.2
N$62: IC4.4(EN) JP8.1 R17.2
N$63: LD4.C R28.2
N$64: Q1.6(B:C) R31.1
N$65: Q1.3(A:C) R28.1
N$66: C22.1 J12.1(V) JP6.3
N$67: Q1.2(B:B) R25.2
N$69: Q1.5(A:B) R23.2
N$71: BTN2.1A BTN2.2A R29.2 R32.2
N$72: BTN1.1A BTN1.2A R27.2 R30.2
PGED1/AN0/RPB0/RB0: JP8.2 ; also sheet 3,4
RPD10/SCK4/RD10: IC3.34(SCK) ; also sheet 5
SQICS0/RPD4/RD4: R24.1 ; also sheet 5
USB_D+: J11.3(D+) J12.3(D+) ; also sheet 2
USB_D-: J11.2(D-) J12.2(D-) ; also sheet 2
USBID/RPF3/RF3: J11.4(ID) ; also sheet 5
VBUS: IC4.1(OUT) J11.1(V) JP6.2 ; also sheet 2,7
VCC3V3: BTN1.1B BTN1.2B BTN2.1B BTN2.2B C21.1 C23.1 C25.1 C26.1 C27.1 IC3.17(VDD) IC3.29(VDD) J13.4(VDD) LD1.A LD2.A LD3.A LD4.A R14.2 R16.2 R18.2 R19.2 R20.2 R21.2 R22.2 ; also sheet 2,4,5,7
VCC5V0: IC4.5(IN) ; also sheet 2,7
Unconnected: IC3.3(JTAG_TDO) IC3.4(JTAG_TCK) IC3.5(JTAG_TMS) IC3.6(JTAG_TDI) IC3.9(JTAG_RST) IC3.21(JTAG_EN) IC3.27(DEBUG_TX) J13.1(DAT2/RSV) J13.8(DAT1/RSV)

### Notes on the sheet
- No Load
- No Load
- MRF24WG0MA
- uSD Connector
- TPS2051BDBVR
- chipKIT WiFire
- Copyright 2014, Digilent Inc.
- KRV
- WiFi, USB, SD Card | CLG/KRV
- B.0
- 500-302 | 03/18/2014

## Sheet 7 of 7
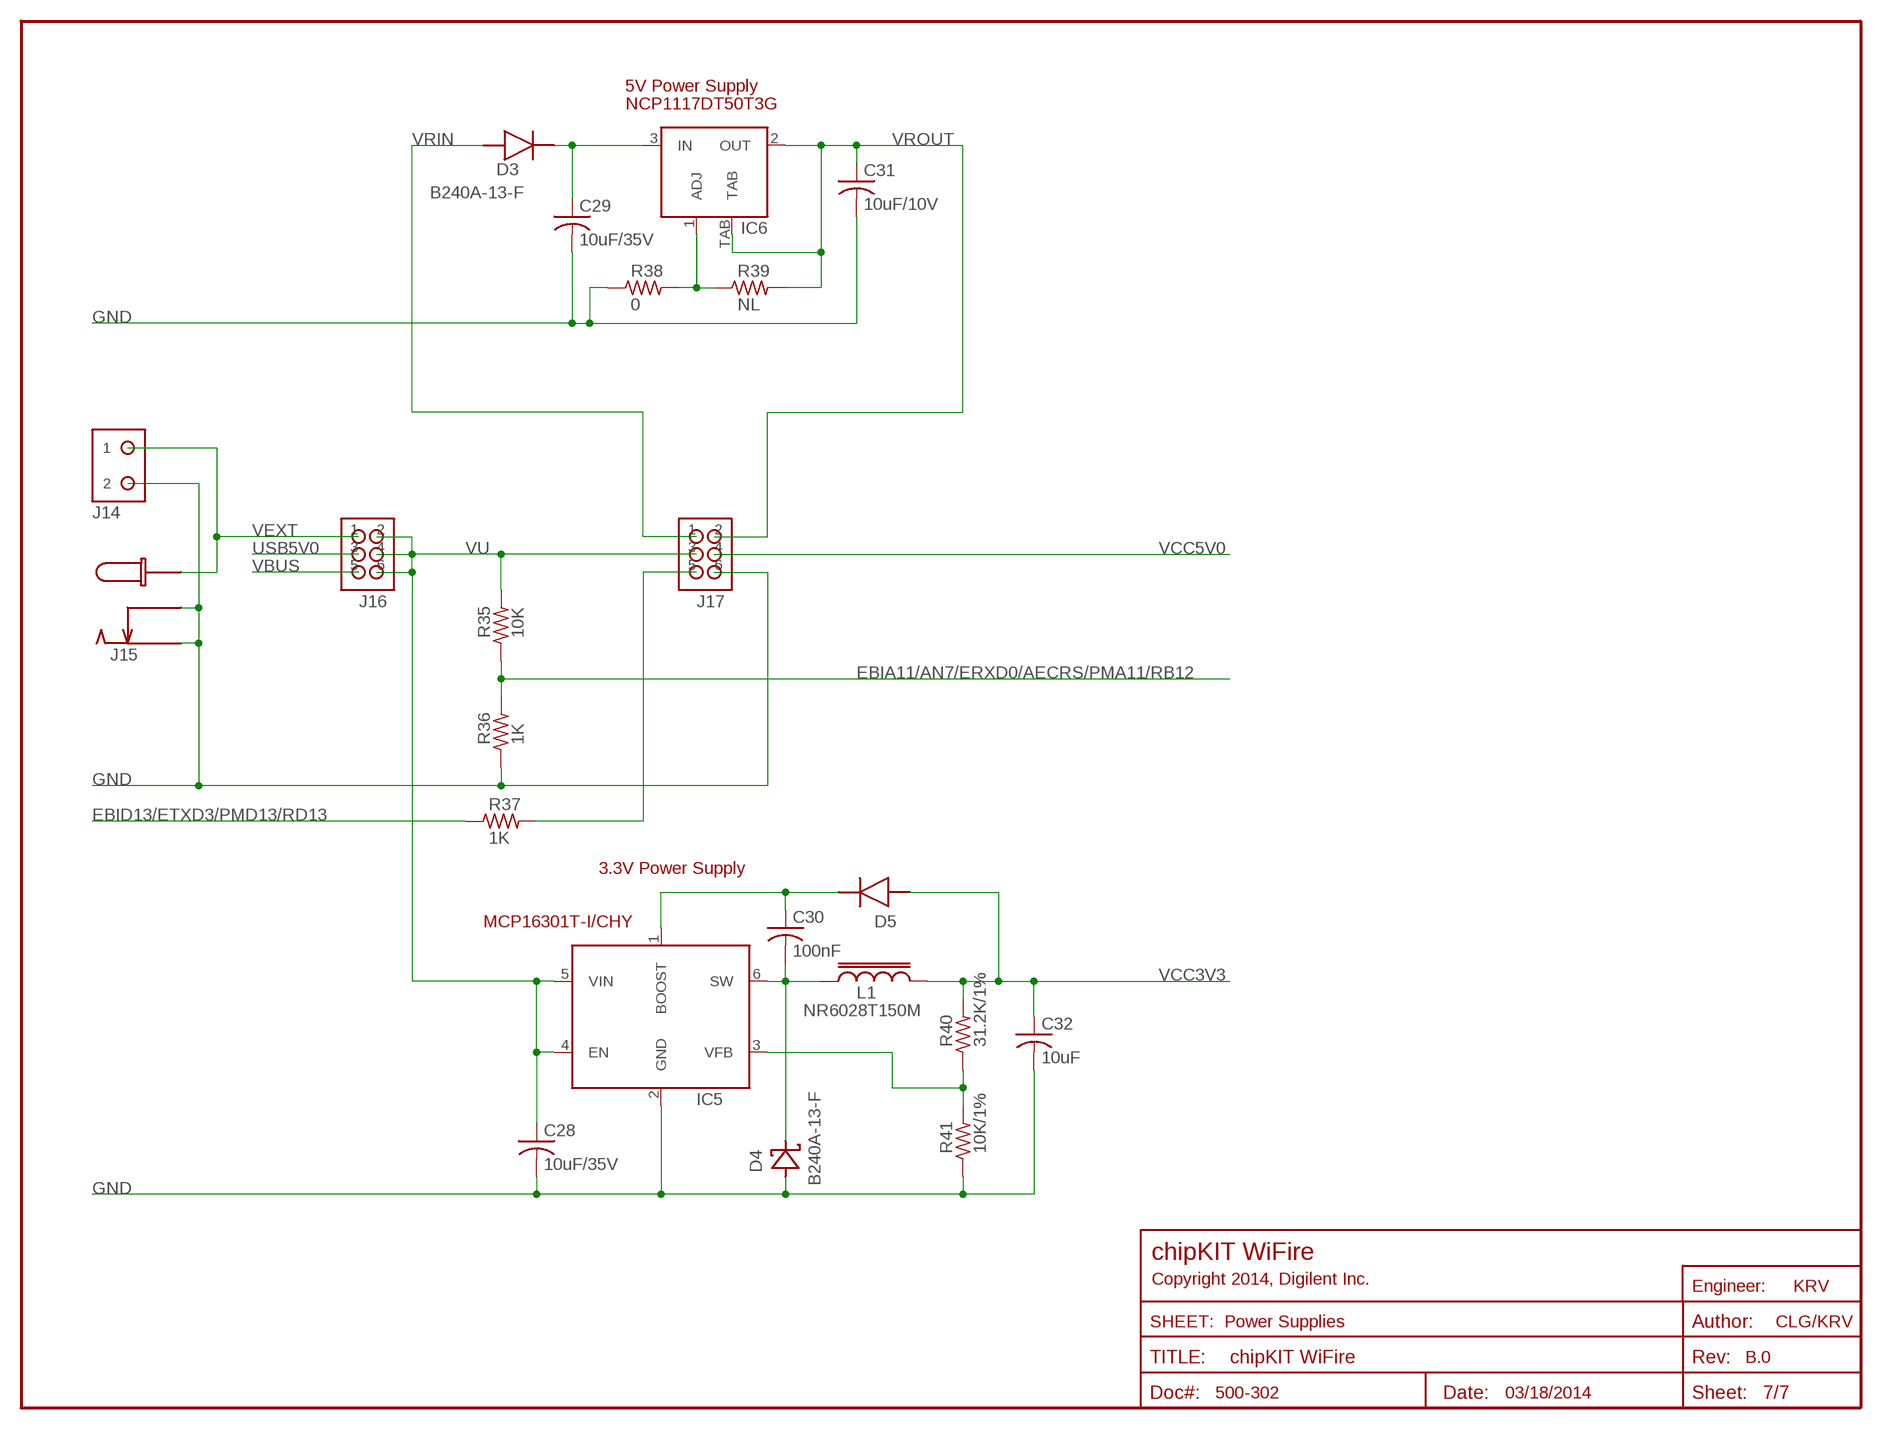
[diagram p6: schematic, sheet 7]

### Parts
C28  10uF/35V  CAP-S1206S  [C1206S]
C29  10uF/35V  CAP-S1206S  [C1206S]
C30  100nF  CAP-S0402S  [C0402S]
C31  10uF/10V  CAP-S0805S  [C0805S]
C32  10uF  CAP-S0805S  [C0805S]
D3  B240A-13-F  DIODESMA  [SMA]
D4  B240A-13-F  SCHOTTKY-SMA  [SMA]
D5  CDSU4148  DIODE0603S  [D0603S]
IC5  MCP16301T-I/CHY  MCP16301  [SOT23-6-CH]
IC6  NCP1117DT50T3G  LM1117MP  [SOT223]
J14  ST. Male  HDR-1X2  [HDR-1X2]
J15  CON-COAX-KLD0202-S  [KLD-0202S]
J16  ST. Male  JPR-2X3  [HDR-2X3]
J17  ST. Male  JPR-2X3  [HDR-2X3]
L1  NR6028T150M  IND-NR6028  [NR60XX]
R35  10K  RES-S0402S  [R0402S]
R36  1K  RES-S0402S  [R0402S]
R37  1K  RES-S0402S  [R0402S]
R38  0  RES-S0603S  [R0603S]
R39  NL  RES-S0402S  [R0402S]
R40  31.2K/1%  RES-S0402S  [R0402S]
R41  10K/1%  RES-S0402S  [R0402S]

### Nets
EBIA11/AN7/ERXD0/AECRS/PMA11/RB12: R35.1 R36.2 ; also sheet 4
EBID13/ETXD3/PMD13/RD13: R37.1 ; also sheet 5
GND: C28.2 C29.2 C31.2 C32.2 D4.A IC5.2(GND) J14.2 J15.2 J15.3 J17.6 R36.1 R38.1 R41.1 ; also sheet 2,3,4,5,6
N$30: J17.5 R37.2
N$34: C30.2 D4.C IC5.6(SW) L1.1
N$35: C30.1 D5.C IC5.1(BOOST)
N$36: IC6.1(ADJ) R38.2 R39.1
N$38: IC5.3(VFB) R40.1 R41.2
N$39: C29.1 D3.C IC6.3(IN)
USB5V0: J16.3 ; also sheet 2
VBUS: J16.5 ; also sheet 2,6
VCC3V3: C32.1 D5.A L1.2 R40.2 ; also sheet 2,4,5,6
VCC5V0: J17.4 ; also sheet 2,6
VEXT: J14.1 J15.1 J16.1 ; also sheet 2
VRIN: D3.A J17.1
VROUT: C31.1 IC6.2(OUT) IC6.TAB J17.2 R39.2
VU: C28.1 IC5.4(EN) IC5.5(VIN) J16.2 J16.4 J16.6 J17.3 R35.2

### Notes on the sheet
- 5V Power Supply
- NCP1117DT50T3G
- 3.3V Power Supply
- chipKIT WiFire
- Copyright 2014, Digilent Inc.
- KRV
- Power Supplies | CLG/KRV
- B.0
- 500-302 | 03/18/2014

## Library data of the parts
BTN1-BTN3 = Mechanical:SW-P8008: 153-000: SPST, Push button, momentary
C1-C17 C19-C32 = Discrete:CAP: Capacitor
D1 = Discrete:BAV99W: BAV99W Dual Surface Mount Switching Diode
D2 = Discrete:NSQA6V8: Low Capacitance Quad ESD Protection Array
D3 D5 = Discrete:DIODE: Diode
D4 = Discrete:SCHOTTKY: Generic Schotkey diode
IC1 = Microchip:PIC32MZ*ECX100: PIC32MZ Embedded Connectivity (EC) Family Microcontroller - 100-pin packages
IC2 = IC:FT232R: FTDI USB UART Serial Converter
IC3 = Microchip:MRF24WB0MA: 2.4 GHz, IEEE Std. 802.11b RF Tranciver Module
IC4 = TI:TPS2041B: Current Limited, Power Distribution Switch
IC5 = Microchip:MCP16301: Microchip MCP16301 High Voltage Input Integrated Switch Step-Down Regulator 600mA, 2 -15V Out, 4-30V In
IC6 = IC:LM1117: LM1117 Adjustable voltage regulator, 1.2V dropout
IC7 = IC:DSC1033: Discera 3.3V PureSilicon Oscillator
J1 = Mechanical:USB-AB-MINI: Kycon KMAB-SMT-5S Mini USB AB type connector
J2 J3 = Mechanical:HDR-1X1
J4 = Mechanical:HDR-1X4
J5 = Mechanical:HDR-1X8
J6 J14 = Mechanical:HDR-1X2
J7 J10 = Mechanical:HDR-2X8: 100mil 2x8 header
J8 = Mechanical:HDR-2X6: 2x6 header with 42mil holes and 100mil spacing
J9 = Mechanical:HDR-2X3
J11 = Mechanical:USB-AB-MICRO
J12 = Mechanical:USB-A: Kycon KUSB-AS-1 USB Type A connector
J13 = Mechanical:2908-05WB-MG: 3M Card Connector microSD
J15 = Mechanical:CON-COAX: COAX Power Connector
J16 J17 = Mechanical:JPR-2X3: Jumper Block: 2x3
JP1 JP3 JP4 = Mechanical:HDR-1X6-OFFSET: 42 mil hole pattern with 16mil offset for jtag connector
JP2 JP5 JP7 JP8 = Mechanical:JPR-1X2
JP6 JP9 = Mechanical:JPR-1X3
L1 = Discrete:IND: Inductors
LD1-LD6 = Discrete:LED: Discrete LED
LOGO1 = Logo:DIGILENT_INC
LOGO2 = Logo:CE: European Union CE Logo
LOGO3 = Logo:WEEE: WEEE Symbol
LOGO4 = Logo:ROHS-CHINA: Chinese ROHS symbol logo
Q1 Q2 = Discrete:MBT3904DW1T1: On-Semiconductor MBT3904DW1T1 Dual General Purpose Transistors
R1-R11 R13-R41 = Discrete:RES: Resistor
U$1 = Logo:CHIPKIT_WIFIRE_LOGO
VR1 = Discrete:POT
X2 = Discrete:XTAL: Quartz Crystal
